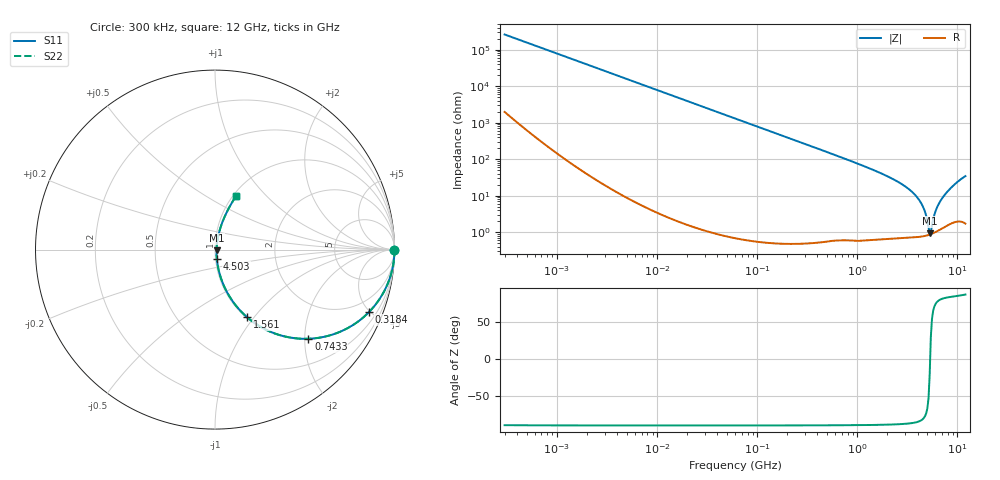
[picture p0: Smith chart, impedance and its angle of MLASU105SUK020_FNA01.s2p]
! MLASU105SUK020_FNA01  S-PARAMETER MODEL  ( General Type )
! Model Generated by TAIYO YUDEN Corporation (http://www.ty-top.com)
! Version 2.0
! TAIYO YUDEN Control No. 120810
! Copyright(c) 2011 TAIYO YUDEN CO.,LTD. All Rights Reserved.
! Product Description (link to TY-COMPAS)
! https://ds.yuden.co.jp/TYCOMPAS/or/detail?pn=MLASU105SUK020CFNA01&u=M
! Products Name : Multilayer Ceramic Capacitors
! Characteristics :
!  Capacitance : 2 pF , Rated Voltage : 50V , TCC : UK / U2K
!  Case Size : 1.0 x 0.5 / 0.039 x 0.02 [mm/inch] , Thickness : 0.5 / 0.02 [mm/inch]
!  (Conditions: Temperature = 25 degC , DC Bias Current/Voltage = 0A / 0V)
! External Node Assignments :
!  1  o---| |---o  2
! GND o---------o GND
! Frequency Range : 0.3MHz  -  12000MHz  [ 401 STEP ]
# MHz S RI R 50
! Freq[MHz].  S11 Real  S11 Imag  S21 Real  S21 Imag  S12 Real  S12 Imag  S22 Real  S22 Imag
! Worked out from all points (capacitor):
!   401 points, 300 kHz to 12 GHz, reference 50 ohm
!   read as one part in series: C = 2.01 pF near 316.3 kHz
!   lowest |Z| = 919 mohm at 5.279 GHz (marker M1)
!   series resonance near 5.335 GHz, so ESL is about 440 pH
!   S11 on the Smith chart (normalised r, x): 300 kHz: open; 318.4 MHz: 1.01, -4.95; 743.3 MHz: 1.01, -2.09; 1.561 GHz: 1.01, -0.93; 4.503 GHz: 1.02, -0.10; 12 GHz: 1.03, +0.69
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0.3  1 -0.00038  3e-06 0.00038  3e-06 0.00038  1 -0.00038
1.769972  1 -0.00224  7.44e-06 0.00224  7.44e-06 0.00224  1 -0.00224
10.44266  0.9998 -0.0132  0.00018 0.0132  0.00018 0.0132  0.9998 -0.0132
60  0.9942 -0.0755  0.00577 0.0755  0.00577 0.0755  0.9942 -0.0755
164.1901  0.9584 -0.1993  0.0416 0.1993  0.0416 0.1993  0.9584 -0.1993
318.4019  0.859 -0.347  0.141 0.347  0.141 0.347  0.859 -0.347
353.9943  0.8311 -0.3735  0.1689 0.3735  0.1689 0.3735  0.8311 -0.3735
743.2595  0.5208 -0.4967  0.4792 0.4967  0.4792 0.4967  0.5208 -0.4967
1048.836  0.3453 -0.4715  0.6547 0.4715  0.6547 0.4715  0.3453 -0.4715
1560.575  0.1799 -0.3774  0.8201 0.3774  0.8201 0.3774  0.1799 -0.3774
2088.533  0.098 -0.2872  0.902 0.2872  0.902 0.2872  0.098 -0.2872
3454.93  0.0241 -0.1288  0.9759 0.1288  0.9759 0.1288  0.0241 -0.1288
4050.141  0.014 -0.0811  0.986 0.0811  0.986 0.0811  0.014 -0.0811
4502.883  0.0101 -0.0497  0.9899 0.0497  0.9899 0.0497  0.0101 -0.0497
4747.894  0.00899 -0.0342  0.991 0.0342  0.991 0.0342  0.00899 -0.0342
5140.631  0.00841 -0.011  0.9916 0.011  0.9916 0.011  0.00841 -0.011
5278.635  0.00851 -0.00328  0.9915 0.00328  0.9915 0.00328  0.00851 -0.00328
5565.855  0.00913 0.0123  0.9909 -0.0123  0.9909 -0.0123  0.00913 0.0123
6188.031  0.0121 0.0424  0.9879 -0.0424  0.9879 -0.0424  0.0121 0.0424
7064.448  0.0195 0.0828  0.9805 -0.0828  0.9805 -0.0828  0.0195 0.0828
9207.246  0.0527 0.181  0.9473 -0.181  0.9473 -0.181  0.0527 0.181
12000  0.1175 0.2981  0.8825 -0.2981  0.8825 -0.2981  0.1175 0.2981
